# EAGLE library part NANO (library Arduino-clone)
Arduino Nano PGS Edit
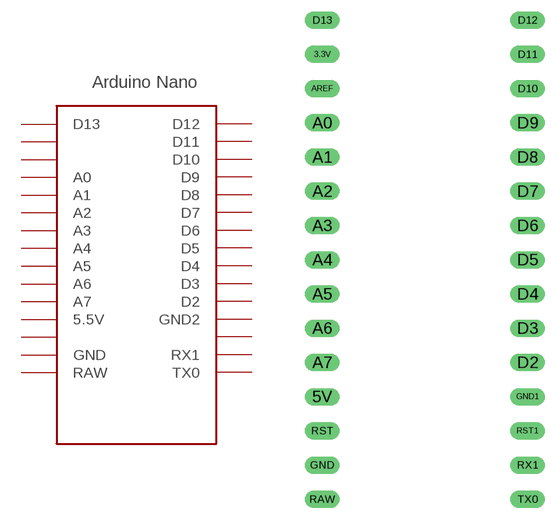
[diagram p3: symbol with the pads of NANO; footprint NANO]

Designator prefix C

## NANOA  [NANO]
3.3V  3.3V  nc
5V  5.5V
A0  A0
A1  A1
A2  A2
A3  A3
A4  A4
A5  A5
A6  A6
A7  A7
AREF  AREF
D2  D2
D3  D3
D4  D4
D5  D5
D6  D6
D7  D7
D8  D8
D9  D9
D10  D10
D11  D11
D12  D12
D13  D13
GND  GND
GND1  GND2
RAW  RAW
RST  0
RST1  RST1
RX1  RX1
TX0  TX0

## NANOB  [NANO]
Pads as for NANO

## NANOC  [NANO]
5V  5.5V
A0  A0
A1  A1
A2  A2
A3  A3
A4  A4
A5  A5
A6  A6
A7  A7
D2  D2
D3  D3
D4  D4
D5  D5
D6  D6
D7  D7
D8  D8
D9  D9
D10  D10
D11  D11
D12  D12
D13  D13
GND  GND
GND1  GND2
RAW  RAW
RX1  RX1
TX0  TX0

## Footprint NANO (pad centres in mm)
drill 0.8 long: 3.3V -10.16,24.13; 5V -10.16,-1.27; A0 -10.16,19.05; A1 -10.16,16.51; A2 -10.16,13.97; A3 -10.16,11.43; A4 -10.16,8.89; A5 -10.16,6.35; A6 -10.16,3.81; A7 -10.16,1.27; AREF -10.16,21.59; D2 5.08,1.27; D3 5.08,3.81; D4 5.08,6.35; D5 5.08,8.89; D6 5.08,11.43; D7 5.08,13.97; D8 5.08,16.51; D9 5.08,19.05; D10 5.08,21.59; D11 5.08,24.13; D12 5.08,26.67; D13 -10.16,26.67; GND -10.16,-6.35; GND1 5.08,-1.27; RAW -10.16,-8.89; RST -10.16,-3.81; RST1 5.08,-3.81; RX1 5.08,-6.35; TX0 5.08,-8.89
